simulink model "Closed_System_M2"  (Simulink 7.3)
settings: Solver=ode45  StartTime=0.0  StopTime=200  RelTol=1e-3
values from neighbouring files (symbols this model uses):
  Cza = -0.032    [init.m]    (also in init_pitch.m)
  Czde = -0.0087    [init.m]    (also in init_pitch.m)
  d2r = 1/r2d    (= 0.0174532925199)    [init.m]    (also in freq.m; frequ.m; init_lat.m; pl.m)
  Mv = 1219.1    [init.m]    (also in init_lat.m; init_pitch.m)
  Qbar = 1220.6    [init.m]    (also in init_lat.m; init_pitch.m)
  r2d = 180/pi    (= 57.2957795131)    [init.m]    (also in freq.m; frequ.m; init_lat.m; pl.m)
  Sref = 145.4    [init.m]    (also in init_lat.m; init_pitch.m)
undefined symbols (not defined in the file or in its folder): Ap2, Bp2, Cp2, Dp2

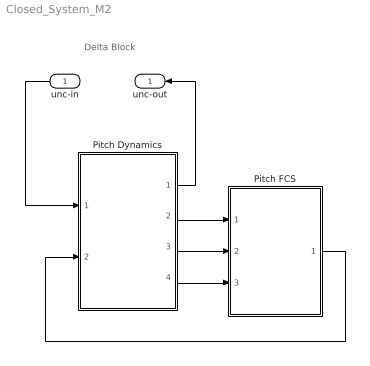
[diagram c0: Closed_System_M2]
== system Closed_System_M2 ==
  note: Delta Block
  unc-in : Inport
  Pitch Dynamics : Subsystem
  Pitch FCS : Subsystem
  unc-out : Outport
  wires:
  Pitch Dynamics/3(q) -> Pitch FCS/2(q)
  Pitch Dynamics/4(Nz) -> Pitch FCS/3(Nz)
  Pitch Dynamics/2(gamma) -> Pitch FCS/1(gamerr)
  Pitch FCS/1(d-elev) -> Pitch Dynamics/2(elev)
  unc-in/1 -> Pitch Dynamics/1(unc-in)
  Pitch Dynamics/1(unc-out) -> unc-out/1

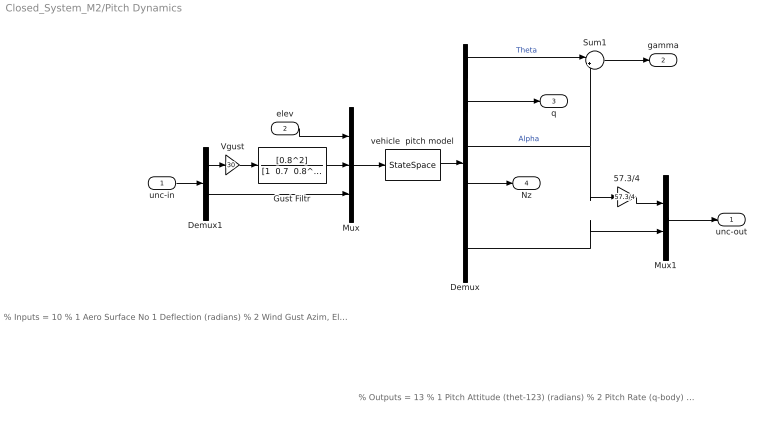
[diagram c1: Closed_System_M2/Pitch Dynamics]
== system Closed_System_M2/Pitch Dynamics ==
  note: % Inputs = 10 % 1 Aero Surface No 1 Deflection (radians) % 2 Wind Gust Azim, Elev Angles=( 45.0 90.0) (deg) % 3 Cm_alpha : -27.273 % Variation % 4 Cz_alpha : -12.500 % Variation % 5 Cm_0 : -27.027 % Variation % 6 CZ_0 : -50.000 % Variation % 7 I_yy : 2.418 % Variation % 8 Xcg locat: 1.909 % Variation % 9 Cz_surf 1: -28.736 % Variation % 10 Cm_surf 1: -20.833 % Variation
  note: % Outputs = 13 % 1 Pitch Attitude (thet-123) (radians) % 2 Pitch Rate (q-body) (rad/sec) % 3 Angle of attack, alfa, (radians) % 4 Accelerom # 2, (along Z), (ft/sec^2) Translat. Acceler % 5 Alpha Sensed at Vane # 1 (radian) % 6 Cm_alpha : -27.273 % Variation % 7 Cz_alpha : -12.500 % Variation % 8 Cm_0 : -27.027 % Variation % 9 CZ_0 : -50.000 % Variation % 10 I_yy : 2.418 % Variation % 11 Xcg locat: 1.909 % Variation % 12 Cz_surf 1: -28.736 % Variation % 13 Cm_surf 1: -20.833 % Variation
  unc-in : Inport
  elev : Inport  Port=2
  57.3/4 : Gain  Gain=57.3/4  ParameterDataType=fixdt(1, 16)  ParameterScaling=2^0  OutDataType=fixdt(1, 16)  OutScaling=2^0
  Demux : Demux  Outputs="[1,1,1,1,1,  8]"
  Demux1 : Demux  Outputs=[1,8]
  Gust Filtr : TransferFcn  Numerator=[0.8^2]  Denominator="[1  0.7  0.8^2]"
  Mux : Mux  Inputs=[1, 1, 8]
  Mux1 : Mux  Inputs="[1,  8]"
  Sum1 : Sum  Inputs=|+-  OutDataType=fixdt(1, 16)  OutScaling=2^0
  Vgust : Gain  Gain=30  ParameterDataType=fixdt(1, 16)  ParameterScaling=2^0  OutDataType=fixdt(1, 16)  OutScaling=2^0
  vehicle  pitch model : StateSpace  A=Ap2  B=Bp2  C=Cp2  D=Dp2
  unc-out : Outport
  gamma : Outport  Port=2
  q : Outport  Port=3
  Nz : Outport  Port=4
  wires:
  vehicle  pitch model/1 -> Demux/1
  Mux/1 -> vehicle  pitch model/1
  Demux/2 -> q/1
  elev/1 -> Mux/1
  Demux/4 -> Nz/1
  Sum1/1 -> gamma/1
  Demux/1 -> Sum1/1  "Theta"
  Gust Filtr/1 -> Mux/2
  Demux/3 -> Sum1/2, 57.3/4/1  "Alpha"
  Demux/6 -> Mux1/2
  Mux1/1 -> unc-out/1
  unc-in/1 -> Demux1/1
  Demux1/1 -> Vgust/1
  Demux1/2 -> Mux/3
  Vgust/1 -> Gust Filtr/1
  57.3/4/1 -> Mux1/1

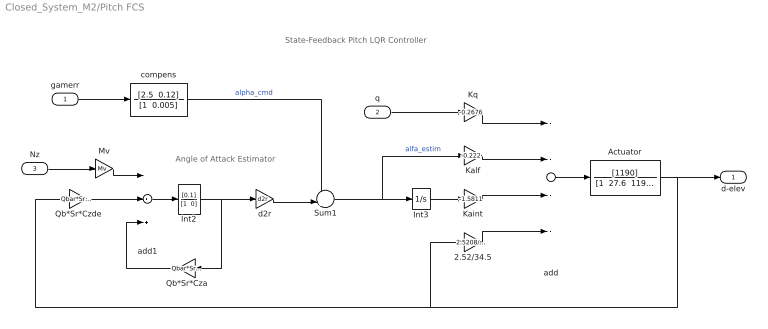
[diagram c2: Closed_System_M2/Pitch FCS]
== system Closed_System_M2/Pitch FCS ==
  note: Angle of Attack Estimator
  note: State-Feedback Pitch LQR Controller
  gamerr : Inport
  q : Inport  Port=2
  Nz : Inport  Port=3
  2.52/34.5 : Gain  Gain=2.5208/34.5  ParameterDataType=fixdt(1, 16)  ParameterScaling=2^0  OutDataType=fixdt(1, 16)  OutScaling=2^0
  Actuator : TransferFcn  Numerator=[1190]  Denominator="[1  27.6  1190]"
  Int2 : TransferFcn  Numerator=[0.1]  Denominator="[1  0]"
  Int3 : Integrator
  Kaint : Gain  Gain=-1.5811  ParameterDataType=fixdt(1, 16)  ParameterScaling=2^0  OutDataType=fixdt(1, 16)  OutScaling=2^0
  Kalf : Gain  Gain=-0.222  ParameterDataType=fixdt(1, 16)  ParameterScaling=2^0  OutDataType=fixdt(1, 16)  OutScaling=2^0
  Kq : Gain  Gain=-0.2676  ParameterDataType=fixdt(1, 16)  ParameterScaling=2^0  OutDataType=fixdt(1, 16)  OutScaling=2^0
  Mv : Gain  Gain=Mv  ParameterDataType=fixdt(1, 16)  ParameterScaling=2^0  OutDataType=fixdt(1, 16)  OutScaling=2^0
  Qb*Sr*Cza : Gain  Gain=Qbar*Sref*Cza  ParameterDataType=fixdt(1, 16)  ParameterScaling=2^0  OutDataType=fixdt(1, 16)  OutScaling=2^0
  Qb*Sr*Czde : Gain  Gain=Qbar*Sref*Czde*r2d  ParameterDataType=fixdt(1, 16)  ParameterScaling=2^0  OutDataType=fixdt(1, 16)  OutScaling=2^0
  Sum1 : Sum  Inputs=++|  OutDataType=fixdt(1, 16)  OutScaling=2^0
  add : Sum  Inputs=----  OutDataType=fixdt(1, 16)  OutScaling=2^-10
  add1 : Sum  Inputs=-++  OutDataType=fixdt(1, 16)  OutScaling=2^-10
  compens : TransferFcn  Numerator="[2.5  0.12]"  Denominator="[1  0.005]"
  d2r : Gain  Gain=d2r  ParameterDataType=fixdt(1, 16)  ParameterScaling=2^0  OutDataType=fixdt(1, 16)  OutScaling=2^0
  d-elev : Outport
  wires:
  d2r/1 -> Sum1/2
  Nz/1 -> Mv/1
  Int2/1 -> Qb*Sr*Cza/1, d2r/1
  Qb*Sr*Czde/1 -> add1/2
  Mv/1 -> add1/1
  Qb*Sr*Cza/1 -> add1/3
  add1/1 -> Int2/1
  gamerr/1 -> compens/1
  compens/1 -> Sum1/1  "alpha_cmd"
  Actuator/1 -> Qb*Sr*Czde/1, 2.52/34.5/1, d-elev/1
  add/1 -> Actuator/1
  q/1 -> Kq/1
  2.52/34.5/1 -> add/4
  Kaint/1 -> add/3
  Int3/1 -> Kaint/1
  Sum1/1 -> Int3/1, Kalf/1  "alfa_estim"
  Kq/1 -> add/1
  Kalf/1 -> add/2
